[IBIS Ver]   4.1
[File Name]   sprm641a.ibs
[File Rev]   1.0
[Date]   April 15, 2013
[Source]   File originated at Texas Instruments
[Copyright]   (c) 2012, Texas Instruments Inc.
[Component]   f771553xpzp
[Manufacturer] Texas Instruments
[Package]
| Variable   Typ   Min   Max
R_pkg   0.244   0.103   0.315
L_pkg   3.95E-09   3.24E-09   4.86E-09
C_pkg   1.36E-12   9.91E-13   2.35E-12
[Pin] signal_name   model_name   R_pin   L_pin   C_pin
1	GPIO11	BCF183350CSHYPBFZ	2.94E-01	4.61E-09	1.13E-12
2	VDDSFL1833	NC	2.78E-01	4.46E-09	1.39E-12
3	GPIO12	BCF183350CSHYPBFZ	2.64E-01	4.25E-09	1.36E-12
4	GPIO13	BCF183350CSHYPBFZ	2.54E-01	4.01E-09	1.33E-12
5	GPIO14	BCF183350CSHYPBFZ	2.46E-01	3.94E-09	1.30E-12
6	GPIO15	BCF183350CSHYPBFZ	2.41E-01	3.83E-09	1.27E-12
7	GPIO16	BCF183350CSHYPBFZ	2.38E-01	3.78E-09	1.25E-12
8	GPIO17	BCF183350CSHYPBFZ	2.37E-01	3.67E-09	1.24E-12
9	GPIO18	BCF183350CSHYPBFZ	2.40E-01	3.74E-09	1.22E-12
10	VDDSFL1833	NC	2.44E-01	3.69E-09	1.21E-12
11	GPIO19	BCF183350CSHYPBFZ	2.50E-01	3.80E-09	1.22E-12
12	GPIO20	BCF183350CSHYPBFZ	2.59E-01	3.88E-09	1.24E-12
13	GPIO21	BCF183350CSHYPBFZ	2.69E-01	4.05E-09	1.24E-12
14	VPP	NC	1.47E-01	3.53E-09	1.53E-12
15	VDDSFL	NC	2.56E-01	3.91E-09	1.23E-12
16	VDD	NC	2.63E-01	3.93E-09	2.07E-12
17	VSSA	NC	1.39E-01	3.38E-09	1.60E-12
18	VDDA	NC	1.03E-01	3.29E-09	2.22E-12
19	VREFHI1	NC	1.39E-01	3.36E-09	1.75E-12
20	ADCINA5	NC	2.43E-01	3.82E-09	1.29E-12
21	ADCINA4	NC	2.44E-01	3.87E-09	1.30E-12
22	ADCINA3	NC	2.49E-01	3.94E-09	1.32E-12
23	ADCINA2	NC	2.57E-01	4.10E-09	1.35E-12
24	ADCINA1	NC	2.67E-01	4.24E-09	1.37E-12
25	ADCINA0	NC	2.81E-01	4.43E-09	1.10E-12
26	ADCINCAL0	NC	2.76E-01	4.44E-09	1.07E-12
27	ADCINCAL1	NC	2.61E-01	4.28E-09	1.34E-12
28	ADCINB0	NC	2.51E-01	4.11E-09	1.34E-12
29	ADCINB1	NC	2.43E-01	3.94E-09	1.31E-12
30	ADCINB2	NC	2.39E-01	3.81E-09	1.29E-12
31	ADCINB3	NC	2.40E-01	3.76E-09	1.27E-12
32	ADCINB4	NC	2.42E-01	3.71E-09	1.26E-12
33	ADCINB5	NC	2.46E-01	3.70E-09	1.26E-12
34	ADCINB6	NC	2.52E-01	3.73E-09	1.27E-12
35	ADCINB7	NC	2.61E-01	3.97E-09	1.27E-12
36	VSSA	NC	1.50E-01	3.62E-09	1.81E-12
37	VREFHI2	NC	1.54E-01	3.66E-09	1.89E-12
38	VDDA	NC	1.14E-01	3.61E-09	2.35E-12
39	VDD	NC	2.40E-01	3.73E-09	1.13E-12
40	VDDSFL	NC	2.45E-01	3.81E-09	1.15E-12
41	VDD3VFL	NC	1.31E-01	3.24E-09	1.45E-12
42	FLT1	NC	2.29E-01	3.62E-09	1.16E-12
43	FLT2	NC	2.30E-01	3.67E-09	1.18E-12
44	VDDSFL	NC	2.36E-01	3.76E-09	1.26E-12
45	VDD	NC	2.38E-01	3.75E-09	2.07E-12
46	TDI	BCF3335DSHYPBFZ	2.41E-01	3.85E-09	1.29E-12
47	TDO	BCF3335DSHYPBFZ	2.51E-01	4.03E-09	1.33E-12
48	TRSTn	BCF3335CSHYPBFZ	2.59E-01	4.12E-09	1.34E-12
49	TMS	IQ0442FS_40P60P_3X2	2.70E-01	4.25E-09	1.34E-12
50	TCK	IQ0442FS_40P60P_3X2	2.83E-01	4.55E-09	1.10E-12
51	GPIO41	BCF3385DSHYPBFZ	2.50E-01	4.21E-09	9.91E-13
52	GPIO58	BCF3385DSHYPBFZ	2.95E-01	4.70E-09	1.33E-12
53	GPIO59	BCF3335DSHYPBFZ	2.79E-01	4.44E-09	1.33E-12
54	GPIO60	BCF3385DSHYPBFZ	2.64E-01	4.32E-09	1.31E-12
55	VDDSFL	NC	2.54E-01	4.04E-09	1.28E-12
56	GPIO61	BCF3335DSHYPBFZ	2.44E-01	3.85E-09	1.25E-12
57	GPIO62	BCF3385DSHYPBFZ	2.32E-01	3.75E-09	1.24E-12
58	GPIO63	BCF3385DSHYPBFZ	2.20E-01	3.55E-09	1.21E-12
59	GPIO64	BCF3335DSHYPBFZ	2.12E-01	3.42E-09	1.19E-12
60	GPIO65	BCF3385DSHYPBFZ	2.08E-01	3.38E-09	1.16E-12
61	GPIO66	BCF3335DSHYPBFZ	2.07E-01	3.31E-09	1.13E-12
62	VDDSFL	NC	2.11E-01	3.32E-09	1.17E-12
63	VDD	NC	2.07E-01	3.29E-09	1.92E-12
64	VREGENZ	IQ0440FS_3X2_7LM	2.07E-01	3.36E-09	1.18E-12
65	VDDSFL1	NC	2.07E-01	3.33E-09	1.15E-12
66	X2	NC	2.08E-01	3.36E-09	1.16E-12
67	VSS	NC	2.13E-01	3.45E-09	1.17E-12
68	X1	NC	2.21E-01	3.59E-09	1.18E-12
69	XRSn	BQ0491FS_3X2_7LM	2.21E-01	3.58E-09	1.21E-12
70	VDDSFL1	NC	2.29E-01	3.71E-09	1.28E-12
71	VDD	NC	2.37E-01	3.85E-09	2.14E-12
72	VDDSFL2	NC	1.41E-01	3.63E-09	1.72E-12
73	GPIO42	NC	2.48E-01	4.15E-09	1.33E-12
74	GPIO43	NC	2.66E-01	4.34E-09	1.33E-12
75	GPIO69	BCF3385DSHYPBFZ	2.91E-01	4.60E-09	1.07E-12
76	GPIO70	BCF3335DSHYPBFZ	3.04E-01	4.78E-09	1.14E-12
77	GPIO71	BCF3385DSHYPBFZ	2.92E-01	4.57E-09	1.41E-12
78	VDD	NC	2.84E-01	4.48E-09	1.38E-12
79	VDDSFL	NC	2.75E-01	4.24E-09	1.35E-12
80	GPIO72	BCF3335DSHYPBFZ	2.72E-01	4.19E-09	1.33E-12
81	GPIO73	BCF3385DSHYPBFZ	2.70E-01	4.21E-09	1.27E-12
82	GPIO78	BCF3385DSHYPBFZ	2.69E-01	4.06E-09	1.19E-12
83	VDDSFL	NC	2.76E-01	4.14E-09	1.30E-12
84	VDD	NC	2.73E-01	4.07E-09	2.19E-12
85	GPIO84	BCF3385DSHYPBFZ	2.74E-01	4.10E-09	1.26E-12
86	GPIO85	BCF3385DSHYPBFZ	2.71E-01	4.06E-09	1.27E-12
87	GPIO86	BCF3385DSHYPBFZ	2.70E-01	3.97E-09	1.27E-12
88	GPIO87	BCF3385DSHYPBFZ	2.69E-01	3.99E-09	1.24E-12
89	VDD	NC	2.70E-01	4.01E-09	2.18E-12
90	VDDSFL	NC	2.69E-01	4.02E-09	1.27E-12
91	GPIO2	GPIORETV2_NFS	2.64E-01	3.96E-09	1.24E-12
92	GPIO3	GPIORETV2_NFS	2.65E-01	4.01E-09	1.27E-12
93	GPIO4	GPIORETV2_NFS	2.69E-01	4.05E-09	1.26E-12
94	VDDSFL	NC	2.74E-01	4.15E-09	1.31E-12
95	VDD	NC	2.78E-01	4.22E-09	1.77E-12
96	GPIO89	BCF3385DSHYPBFZ	2.84E-01	4.37E-09	1.35E-12
97	GPIO90	BCF3385DSHYPBFZ	2.92E-01	4.53E-09	1.40E-12
98	GPIO91	BCF3385DSHYPBFZ	3.04E-01	4.65E-09	1.40E-12
99	GPIO92	BCF3385DSHYPBFZ	3.15E-01	4.86E-09	1.37E-12
100	GPIO10	BCF183350CSHYPBFZ	3.01E-01	4.65E-09	1.11E-12
| End of package information
|   Component BCF3335DSHYPBFZ
[Component]   BCF3335DSHYPBFZ
[Manufacturer]   Texas Instruments
[Package]
|  variable   typ   min   max
R_pkg   0   0   0
L_pkg   0   0   0
C_pkg   0   0   0
[Pin]   signal_name   model_name   R_pin   L_pin   C_pin
VSS   VSS   GND
VDDS   VDDS   POWER
PAD   PAD   BCF3335DSHYPBFZ
[Model Selector] BCF3335DSHYPBFZ
BCF3335D_WK_PU_ON  Cell operated at 3.3(nom)
|BCF3335D_WK_PU_ON; WEAK_PULLUP_ON
BCF3335D_DRIVER_MODE  Cell operated at 3.3(nom)
|BCF3335D_DRIVER_MODE
BCF3335D_WK_PD_ON  Cell operated at 3.3(nom)
|   Component BCF3385DSHYPBFZ
[Component]   BCF3385DSHYPBFZ
[Manufacturer]   Texas Instruments
[Package]
|  variable   typ   min   max
R_pkg   0   0   0
L_pkg   0   0   0
C_pkg   0   0   0
[Pin]   signal_name   model_name   R_pin   L_pin   C_pin
VSS   VSS   GND
VDDS   VDDS   POWER
PAD   PAD   BCF3385DSHYPBFZ
[Model Selector] BCF3385DSHYPBFZ
BCF3385D_WK_PU_ON  Cell operated at 3.3(nom)
|BCF3385D_WK_PU_ON; WEAK_PULLUP_ON
BCF3385D_DRIVER_MODE  Cell operated at 3.3(nom)
|BCF3385D_DRIVER_MODE
BCF3385D_WK_PD_ON  Cell operated at 3.3(nom)
|   Component BCF183350CSHYPBFZ
[Component]   BCF183350CSHYPBFZ
[Manufacturer]   Texas Instruments
[Package]
|  variable   typ   min   max
R_pkg   0   0   0
L_pkg   0   0   0
C_pkg   0   0   0
[Pin]   signal_name   model_name   R_pin   L_pin   C_pin
VSS   VSS   GND
VDDS   VDDS   POWER
PAD   PAD   BCF183350CSHYPBFZ
[Model Selector] BCF183350CSHYPBFZ
BCF183350C_WK_PU_ON  Cell operated at 3.3(nom)
|BCF183350C_WK_PU_ON; WEAK_PULLUP_ON
BCF183350C_DRIVER_MODE  Cell operated at 3.3(nom)
|BCF183350C_DRIVER_MODE
BCF183350C_WK_PD_ON  Cell operated at 3.3(nom)
|BCF183350C_WK_PD_ON; WEAK_PULLDOWN_ON
WK_PU_ON_1P8  Cell operated at 1.8(nom)
|WK_PU_ON_1P8; WEAK_PULLUP_ON
DRIVER_MODE_1P8  Cell operated at 1.8(nom)
|DRIVER_MODE_1P8
WK_PD_ON_1P8  Cell operated at 1.8(nom)
|   Component IQ0442FS_40P60P_3X2
[Component]   IQ0442FS_40P60P_3X2
[Manufacturer]   Texas Instruments
[Package]
|  variable   typ   min   max
R_pkg   0   0   0
L_pkg   0   0   0
C_pkg   0   0   0
[Pin]   signal_name   model_name   R_pin   L_pin   C_pin
VSS   VSS   GND
VDDS   VDDS   POWER
PAD   PAD   IQ0442FS_40P60P_3X2
[Model Selector] IQ0442FS_40P60P_3X2
S_40P60P_3X2_7LM_3P3  Cell operated at 3.3(nom)
|IQ0442FS_40P60P_3X2_3P3; PUPD_OFF
0P60P_3X2_7LM_PU_3P3  Cell operated at 3.3(nom)
|IQ0442FS_40P60P_3X2_PU_3P3; PULLUP_ON
0P60P_3X2_7LM_PD_3P3  Cell operated at 3.3(nom)
|   Component IQ0440FS_3X2_7LM
[Component]   IQ0440FS_3X2_7LM
[Manufacturer]   Texas Instruments
[Package]
|  variable   typ   min   max
R_pkg   0   0   0
L_pkg   0   0   0
C_pkg   0   0   0
[Pin]   signal_name   model_name   R_pin   L_pin   C_pin
VSS   VSS   GND
VDDS   VDDS   POWER
PAD   PAD   IQ0440FS_3X2_7LM
[Model Selector] IQ0440FS_3X2_7LM
440FS_3X2_7LM_PD_3P3  Cell operated at 3.3(nom)
|IQ0440FS_3X2_7LM_PD_3P3; PULLDOWN_ON
IQ0440FS_3X2_7LM_3P3  Cell operated at 3.3(nom)
|   Component BQ0491FS_3X2_7LM
[Component]   BQ0491FS_3X2_7LM
[Manufacturer]   Texas Instruments
[Package]
|  variable   typ   min   max
R_pkg   0   0   0
L_pkg   0   0   0
C_pkg   0   0   0
[Pin]   signal_name   model_name   R_pin   L_pin   C_pin
VSS   VSS   GND
VDDS   VDDS   POWER
PAD   PAD   BQ0491FS_3X2_7LM
[Model Selector] BQ0491FS_3X2_7LM
491FS_3X2_7LM_PU_3P3  Cell operated at 3.3(nom)
|BQ0491FS_3X2_7LM_PU_3P3; PULLUP_ON
491FS_3X2_7LM_PZ_3P3  Cell operated at 3.3(nom)
|   Component GPIORETV2_NFS
[Component]   GPIORETV2_NFS
[Manufacturer]   Texas Instruments
[Package]
|  variable   typ   min   max
R_pkg   0   0   0
L_pkg   0   0   0
C_pkg   0   0   0
[Pin]   signal_name   model_name   R_pin   L_pin   C_pin
VSS   VSS   GND
VDDS   VDDS   POWER
PAD   PAD   GPIORETV2_NFS
[Model Selector] GPIORETV2_NFS
GPIORET_WK_PD_ON_3P3  Cell operated at 3.3(nom)
|GPIORET_WK_PD_ON_3P3; WEAK_PULLDOWN_ON
RET_8MA_OPEN_DRAIN  Cell operated at 3.3(nom)
|RET_8MA_OPEN_DRAIN; 8MA_OPEN_DRAIN_SLW
RET_DRVR_2MA_PUPDOFF  Cell operated at 3.3(nom)
|RET_DRVR_2MA_PUPDOFF
RET_4MA_OPEN_DRAIN  Cell operated at 3.3(nom)
|RET_4MA_OPEN_DRAIN; 4MA_OPEN_DRAIN
GPIORET_WK_PU_ON_3P3  Cell operated at 3.3(nom)
|GPIORET_WK_PU_ON_3P3; WEAK_PULLUP_ON
RET_2MA_OPEN_DRAIN  Cell operated at 3.3(nom)
|RET_2MA_OPEN_DRAIN; 2MA_OPEN_DRAIN
RET_DRVR_8MA_PUPDOFF  Cell operated at 3.3(nom)
|RET_DRVR_8MA_PUPDOFF
RET_DRVR_MODE_8MA_PUPDOFF_SLEW  Cell operated at 3.3(nom)
|RET_DRVR_MODE_8MA_PUPDOFF_SLEW
RET_DRVR_MODE_4MA_PUPDOFF  Cell operated at 3.3(nom)
|RET_DRVR_MODE_4MA_PUPDOFF
RET_8MA_OPEN_DRAIN_3P3  Cell operated at 3.3(nom)
|   Component BCF3335CSHYPBFZ
[Component]   BCF3335CSHYPBFZ
[Manufacturer]   Texas Instruments
[Package]
|  variable   typ   min   max
R_pkg   0   0   0
L_pkg   0   0   0
C_pkg   0   0   0
[Pin]   signal_name   model_name   R_pin   L_pin   C_pin
VSS   VSS   GND
VDDS   VDDS   POWER
PAD   PAD   BCF3335CSHYPBFZ
[Model Selector] BCF3335CSHYPBFZ
BCF3335C_WK_PU_ON_3P3  Cell operated at 3.3(nom)
|BCF3335C_WK_PU_ON_3P3; WEAK_PULLUP_ON
BCF3335C_DRIVER_MODE_3P3  Cell operated at 3.3(nom)
|BCF3335C_DRIVER_MODE_3P3
BCF3335C_WK_PD_ON_3P3  Cell operated at 3.3(nom)
| Models and submodels in the file (32): BCF3335D_WK_PU_ON (Input), BCF3335D_DRIVER_MODE (I/O), BCF3335D_WK_PD_ON (Input), BCF3385D_WK_PU_ON (Input), BCF3385D_DRIVER_MODE (I/O), BCF3385D_WK_PD_ON (Input), WK_PU_ON_1P8 (Input), DRIVER_MODE_1P8 (I/O), WK_PD_ON_1P8 (Input), BCF183350C_WK_PU_ON (Input), BCF183350C_DRIVER_MODE (I/O), BCF183350C_WK_PD_ON (Input), S_40P60P_3X2_7LM_3P3 (Input), 0P60P_3X2_7LM_PU_3P3 (Input), 0P60P_3X2_7LM_PD_3P3 (Input), 440FS_3X2_7LM_PD_3P3 (Input), IQ0440FS_3X2_7LM_3P3 (Input), 491FS_3X2_7LM_PU_3P3 (I/O), 491FS_3X2_7LM_PZ_3P3 (I/O), GPIORET_WK_PD_ON_3P3 (Input), RET_8MA_OPEN_DRAIN (I/O_open_drain), RET_DRVR_2MA_PUPDOFF (I/O), RET_4MA_OPEN_DRAIN (I/O_open_drain), GPIORET_WK_PU_ON_3P3 (Input), RET_2MA_OPEN_DRAIN (I/O_open_drain), RET_DRVR_8MA_PUPDOFF (I/O), RET_DRVR_MODE_8MA_PUPDOFF_SLEW (I/O), RET_DRVR_MODE_4MA_PUPDOFF (I/O), RET_8MA_OPEN_DRAIN_3P3 (I/O_open_drain), BCF3335C_WK_PU_ON_3P3 (Input), BCF3335C_DRIVER_MODE_3P3 (I/O), BCF3335C_WK_PD_ON_3P3 (Input)
